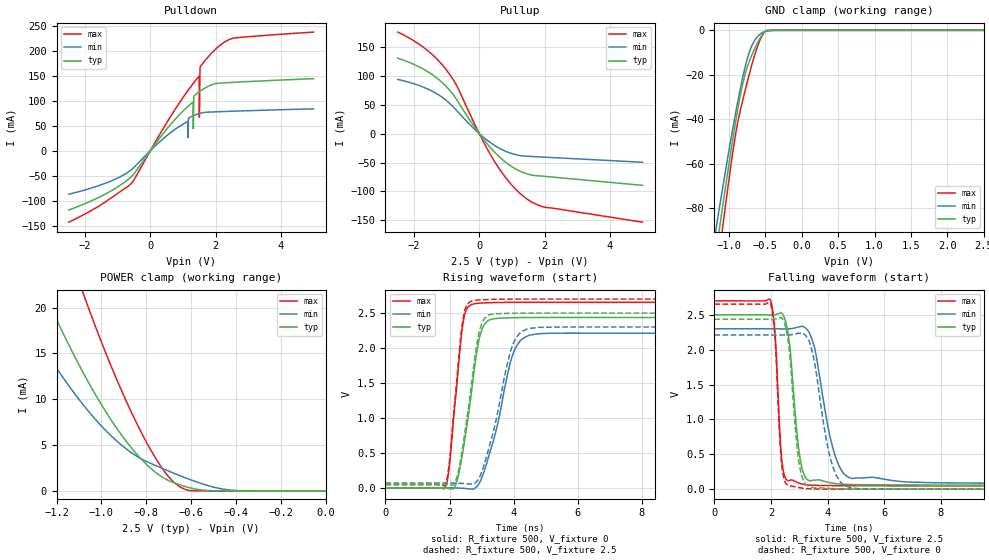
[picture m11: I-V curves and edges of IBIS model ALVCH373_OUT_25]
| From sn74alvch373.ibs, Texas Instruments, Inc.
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[Model]   ALVCH373_OUT_25
Model_type  3-state
Enable   Active-Low
Vref =   0
Rref =   500
Cref =   30p
Vmeas =   1.25
| variable   typ   min   max
C_comp   6.73pF   5.90pF   7.68pF
| C_pullup   8.66pF   6.71pF   9.85pF
| C_pulldown   20.67pF   6.83pF   47.35pF
| C_tri-state   6.73pF   5.90pF   7.68pF
[Temperature Range]   40   100   -40
| Ambient temperature   25   85   -40
[Voltage range]   2.5   2.3   2.7
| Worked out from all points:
|   slope of the pulldown table from 0 to 0.375 V, typ, clamps not added: 11.4 ohm
|   slope of the pullup table from 0 to 0.375 V, typ, clamps not added: 14.2 ohm
|   GND clamp passes 1 mA (typ) near -0.52 V on its own axis
|   POWER clamp passes 1 mA (typ) near -0.69 V on its own axis
|   rising waveform, R_fixture 500, V_fixture 0: 20-80 % time 449ps typ, 669ps min, 314ps max; typ from 0 V to 2.44 V
|   falling waveform, R_fixture 500, V_fixture 2.5: 20-80 % time 316ps typ, 615ps min, 196ps max; typ from 2.5 V to 0.054 V
|   rising waveform, R_fixture 500, V_fixture 2.5: 20-80 % time 441ps typ, 652ps min, 312ps max; typ from 0.054 V to 2.5 V
|   falling waveform, R_fixture 500, V_fixture 0: 20-80 % time 298ps typ, 540ps min, 193ps max; typ from 2.44 V to 0 V
[GND Clamp]
| ALVCH373_OUT_25
|   Voltage   I(typ)   I(min)   I(max)
-2.5V     -430.3mA   -381.4mA   -482.2mA
-1.18V    -100.5mA   -89.65mA   -112.8mA
-1.15V    -93.58mA   -83.54mA   -104.9mA
-1.12V    -86.71mA   -77.49mA   -97.14mA
-1.09V    -79.91mA   -71.51mA   -89.44mA
-1.065V   -74.3mA    -66.57mA   -83.1mA
-910mV    -41.41mA   -37.41mA   -46.92mA
-805mV    -23.23mA   -20.21mA   -30.64mA
-690mV    -11.46mA   -7.21mA    -15.93mA
-540mV    -1.773mA   -971.7uA   -2.146mA
-475mV    -42.56uA   -359uA     -30.01uA
2.5V      99.67pA    107.6nA    13.28pA
[POWER Clamp]
| ALVCH373_OUT_25
|   Voltage   I(typ)   I(min)   I(max)
-2.5V     112.9mA    83.82mA    156.5mA
-1.405V   30.33mA    21.74mA    46.42mA
-1.385V   29.11mA    20.85mA    44.74mA
-1.245V   21.09mA    15.09mA    33.46mA
-1.085V   13.07mA    9.514mA    21.81mA
-1.07V    12.39mA    9.055mA    20.79mA
-860mV    4.505mA    4.065mA    8.248mA
-750mV    1.867mA    2.682mA    3.235mA
-670mV    829.8uA    1.861mA    798.1uA
-605mV    333.4uA    1.24mA     37.9uA
-430mV    1.426uA    104.2uA    31.21nA
-31.15fV  99.67pA    628.4pA    14.82pA
[Pulldown]
| ALVCH373_OUT_25
|   Voltage   I(typ)   I(min)   I(max)
-2.5V     -118.6mA   -87.07mA   -142.9mA
-575mV    -51.47mA   -37.62mA   -64.61mA
1.295V    96.4mA     69.23mA    132.7mA
1.31V     96.95mA    69.67mA    133.9mA
1.315V    43.72mA    69.81mA    134.4mA
1.335V    109.1mA    70.37mA    136.1mA
1.49V     117.3mA    74mA       148.4mA
1.495V    117.6mA    74.09mA    148.6mA
1.5V      117.8mA    74.19mA    66.9mA
1.53V     119.2mA    74.72mA    168.2mA
2.15V     135.1mA    77.94mA    211.3mA
5V        143.8mA    83.55mA    236.9mA
[Pullup]
| ALVCH373_OUT_25
|   Voltage   I(typ)   I(min)   I(max)
-2.5V     131mA      94.16mA    176.4mA
-1.655V   110.2mA    79.39mA    147.4mA
-1.31V    97.07mA    69.54mA    130.2mA
-1.005V   81.43mA    57.45mA    110.4mA
-680mV    57.9mA     39.24mA    82.01mA
30mV      -2.342mA   -1.535mA   -3.449mA
445mV     -30.71mA   -19.54mA   -46.2mA
915mV     -54.12mA   -32.94mA   -83.88mA
1.385V    -68.28mA   -38.94mA   -110.2mA
1.695V    -72.57mA   -39.84mA   -121.3mA
2.005V    -74.04mA   -40.76mA   -127.5mA
5V        -89.66mA   -49.55mA   -153.6mA
[Ramp]
| ALVCH373_OUT_25
| variable   typ   min   max
dV/dt_r   1.47/4.58E-10   1.34/6.79E-10   1.60/3.21E-10
dV/dt_f   1.49/3.24E-10   1.36/6.40E-10   1.61/2.03E-10
R_load = 500
[Rising Waveform]
| ALVCH373_OUT_25
R_fixture =   500
C_fixture =   0
L_fixture =   0
V_fixture =   0
V_fixture_min = 0
V_fixture_max = 0
|   Time   V(typ)   V(min)   V(max)
0s        53.21pV    3.253nV    41.34pV
1.875ns   -3.71mV    993.8uV    19.57mV
1.995ns   -10.95mV   723.7uV    328.6mV
2.175ns   32.42mV    -277.9uV   1.239V
2.42ns    537.6mV    -6.001mV   2.361V
2.8ns     1.796V     -1.608mV   2.635V
3.1ns     2.346V     267.5mV    2.646V
4.005ns   2.434V     1.948V     2.653V
4.735ns   2.437V     2.202V     2.654V
40ns      2.437V     2.212V     2.654V
[Falling Waveform]
| ALVCH373_OUT_25
R_fixture =   500
C_fixture =   0
L_fixture =   0
V_fixture =   2.5
V_fixture_min = 2.3
V_fixture_max = 2.7
|   Time   V(typ)   V(min)   V(max)
0s        2.5V       2.3V       2.7V
1.98ns    2.498V     2.3V       2.712V
2.14ns    2.503V     2.3V       2.24V
2.425ns   2.499V     2.298V     283.2mV
2.64ns    2.131V     2.299V     124.2mV
3.18ns    199.1mV    2.323V     67.24mV
3.55ns    129mV      2.013V     55.23mV
4.25ns    81.35mV    499.5mV    50.81mV
4.85ns    66.32mV    154.8mV    49.66mV
40ns      53.69mV    69.65mV    45.84mV
[Rising Waveform]
| ALVCH373_OUT_25
R_fixture =   500
C_fixture =   0
L_fixture =   0
V_fixture =   2.5
V_fixture_min = 2.3
V_fixture_max = 2.7
|   Time   V(typ)   V(min)   V(max)
0s        53.67mV    69.18mV    45.84mV
1.875ns   49.64mV    69.92mV    66.07mV
1.985ns   43.2mV     69.59mV    338.4mV
2.175ns   88.64mV    68.41mV    1.306V
2.415ns   604.2mV    63.05mV    2.405V
2.79ns    1.872V     68.01mV    2.682V
3.085ns   2.421V     344.4mV    2.691V
3.945ns   2.496V     2.017V     2.7V
4.52ns    2.499V     2.283V     2.7V
40ns      2.5V       2.3V       2.7V
[Falling Waveform]
| ALVCH373_OUT_25
R_fixture =   500
C_fixture =   0
L_fixture =   0
V_fixture =   0
V_fixture_min = 0
V_fixture_max = 0
|   Time   V(typ)   V(min)   V(max)
0s        2.437V     2.212V     2.654V
1.98ns    2.435V     2.212V     2.663V
2.13ns    2.439V     2.211V     2.219V
2.41ns    2.439V     2.21V      243.3mV
2.63ns    2.049V     2.212V     50.99mV
3.04ns    266.6mV    2.237V     18.3mV
3.455ns   24.68mV    1.973V     4.143mV
4.195ns   7.679mV    311mV      452.1uV
4.86ns    1.086mV    15.95mV    152.7uV
40ns      2.258uV    20.48uV    360.9nV
